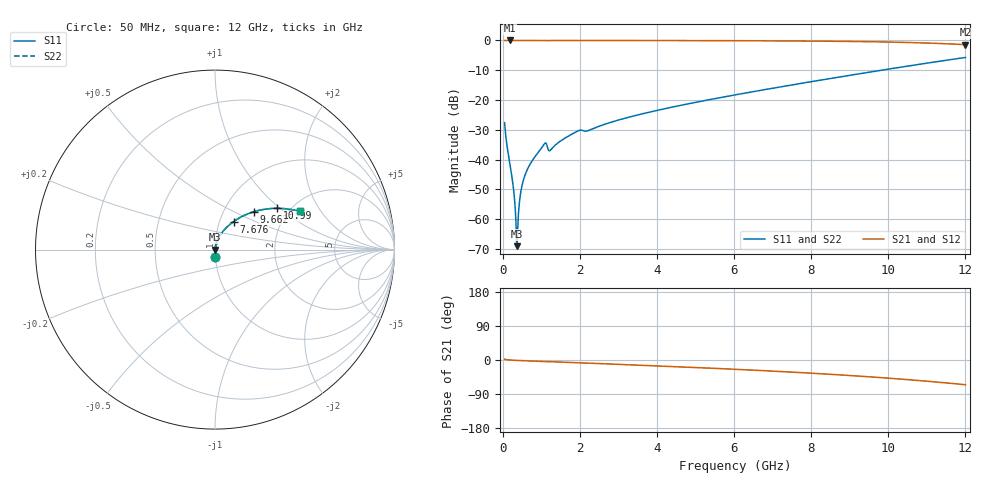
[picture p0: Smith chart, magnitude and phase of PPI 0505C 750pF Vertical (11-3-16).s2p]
# GHz S MA R 50
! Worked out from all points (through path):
!   1601 points, 50 MHz to 12 GHz, reference 50 ohm
!   highest |S21| = 0.00 dB at 199.4 MHz (marker M1); lowest = -1.4 dB at 12 GHz (marker M2)
!   group delay of S21, straight-line fit = 14.4 ps
!   lowest |S11| = -69.1 dB at 371.2 MHz (marker M3), VSWR 1.00, Z = 50 + j0.00546 ohm
!   |S11| at or under -10 dB: start of sweep to 9.822 GHz
!   |S22| runs from -69.1 to -5.7 dB; largest |S21 - S12| = 0
!   S11 on the Smith chart (normalised r, x): 50 MHz: 1.00, -0.08; 7.676 GHz: 1.16, +0.38; 9.662 GHz: 1.38, +0.65; 10.99 GHz: 1.72, +0.96; 12 GHz: 2.26, +1.31
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0.05  0.04159 -87.5  0.9989 2.2  0.9989 2.2  0.04159 -87.5
0.199375  0.007551 -88.0  0.9997 -0.2  0.9997 -0.2  0.007551 -88.0
0.2665938  0.003831 -85.9  0.9997 -0.6  0.9997 -0.6  0.003831 -85.9
0.3338125  0.001212 -75.0  0.9996 -0.9  0.9996 -0.9  0.001212 -75.0
0.3711563  0.000351 8.9  0.9996 -1.1  0.9996 -1.1  0.000351 8.9
0.4085  0.001227 71.8  0.9996 -1.3  0.9996 -1.3  0.001227 71.8
0.46825  0.002813 80.8  0.9996 -1.5  0.9996 -1.5  0.002813 80.8
0.5429375  0.004634 83.2  0.9996 -1.9  0.9996 -1.9  0.004634 83.2
0.6549687  0.007154 84.1  0.9995 -2.3  0.9995 -2.3  0.007154 84.1
0.82675  0.0109 84.0  0.9993 -3.0  0.9993 -3.0  0.0109 84.0
1.080688  0.01829 75.3  0.9964 -4.2  0.9964 -4.2  0.01829 75.3
1.237531  0.01438 73.6  0.9968 -4.4  0.9968 -4.4  0.01438 73.6
1.596031  0.02248 81.5  0.9986 -6.0  0.9986 -6.0  0.02248 81.5
2.044156  0.03109 73.4  0.9946 -7.7  0.9946 -7.7  0.03109 73.4
4.038312  0.06767 73.4  0.9963 -15.7  0.9963 -15.7  0.06767 73.4
6.025  0.1217 64.9  0.9908 -24.5  0.9908 -24.5  0.1217 64.9
7.675594  0.1871 56.5  0.98 -32.9  0.98 -32.9  0.1871 56.5
8.019156  0.2039 54.6  0.9765 -34.9  0.9765 -34.9  0.2039 54.6
9.662281  0.3045 44.1  0.9492 -45.4  0.9492 -45.4  0.3045 44.1
10.01331  0.3309 41.5  0.9402 -48.0  0.9402 -48.0  0.3309 41.5
10.99172  0.415 33.7  0.9056 -55.9  0.9056 -55.9  0.415 33.7
12  0.5175 24.3  0.8504 -65.2  0.8504 -65.2  0.5175 24.3
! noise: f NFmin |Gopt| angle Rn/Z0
0.05  0.0003087  0.8321  0.187  0.0003877
1.372  0.004282  0.6932  3.949  0.002717
2.701  0.005809  0.5841  7.554  0.002537
4.031  0.006985  0.5098  10.84  0.002457
5.36  0.008749  0.4891  14.01  0.002897
6.682  0.01076  0.4864  17.05  0.003516
8.012  0.01316  0.497  20.03  0.004387
9.341  0.01613  0.5195  23  0.005663
10.67  0.02002  0.5538  26.05  0.007652
12  0.02543  0.6002  29.28  0.01101
